(* FB_CylinderTempDiag		- number of control signals控制信号的数量:
									one direction is controllable一个方向是可控的
							- type of feedback signal反馈信号的类型:
									feedback in base and work position基准和工作位置的反馈
							- with temperature diagnosis带温度诊断					*)

FUNCTION_BLOCK FB_CylinderTempDiag EXTENDS FB_CylinderTemp
VAR_INPUT
	fTempMax		AT %I*	: LREAL;						// Global input signal: maximal allowed cylinder temperature for temperature monitoring全局输入信号：用于温度监测的最大允许气缸温度
	fTempMin		AT %I*	: LREAL;						// Global input signal: minimal allowed cylinder temperature for temperature monitoring全局输入信号：用于温度监测的最小允许气缸温度
END_VAR
VAR_OUTPUT
	bError					: BOOL;							// Error signal (diagnosed from temperature monitoring)错误信号（通过温度监测诊断）
	sErrorMsg				: STRING;						// Error message错误消息
END_VAR

// =========================================================
;
// =========================================================

METHOD PROTECTED Diag
VAR_INPUT
END_VAR
// =========================================================
// Error if temperatur of cylinder is not in accepted interval如果气缸温度不在可接受的区间内，则出现错误

	
	bError := NOT (fTempCurrent >= fTempMin AND fTempCurrent <= fTempMax);
	
	IF bError THEN
		IF fTempCurrent > fTempMax THEN
			sErrorMsg := 'Temperature above maximum';
		ELSE
			sErrorMsg := 'Temperature below minimum';
		END_IF
	ELSE
		sErrorMsg := '';
	END_IF

// =========================================================
END_METHOD

METHOD Reset
VAR_INPUT
END_VAR
// =========================================================
	
// Calling method Reset of base class FB_Cylinder via 'SUPER^.'通过'SUPER^'调用FB_Cylinder的方法Reset
SUPER^.Reset();			

// Reset error重置错误
bError 		:= FALSE;
sErrorMsg 	:= '';

// =========================================================
END_METHOD

METHOD PROTECTED StateMachine
VAR_INPUT
	bBasePosReq		: BOOL;
	bWorkPosReq		: BOOL;
END_VAR
// =========================================================

IF NOT bError THEN
	// Calling method StateMachine of base class FB_Cylinder via 'SUPER^.'通过'SUPER^'调用FB_Cylinder的方法StateMachine
	SUPER^.StateMachine(bBasePosReq := bBasePosReq,
						bWorkPosReq	:= bWorkPosReq );
	
	// Diagnosis诊断
	Diag();
END_IF

// =========================================================
END_METHOD

END_FUNCTION_BLOCK
